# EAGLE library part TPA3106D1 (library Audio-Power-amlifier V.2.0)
40-W MONO CLASS-D AUDIO POWER AMPLIFIER
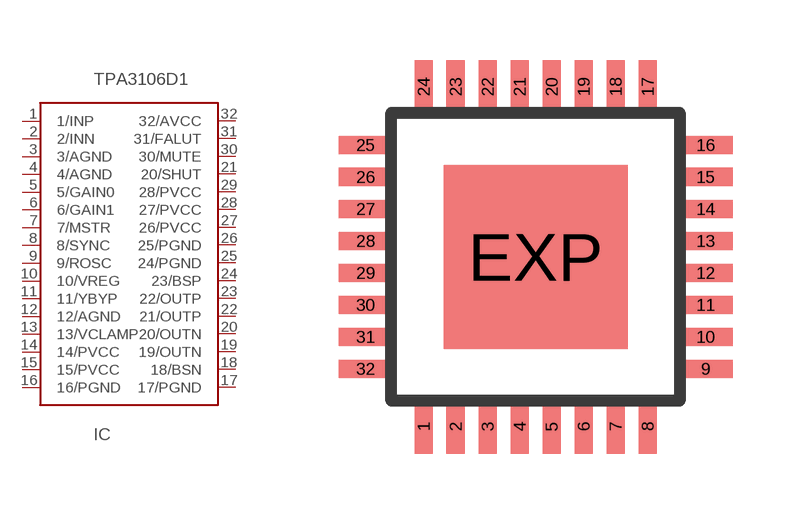
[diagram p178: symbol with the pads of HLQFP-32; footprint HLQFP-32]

Designator prefix IC

## TPA3106D1  [HLQFP-32]
1  1/INP  in
2  2/INN  in
3  3/AGND  pwr
4  4/AGND  pwr
5  5/GAIN0  in
6  6/GAIN1  in
7  7/MSTR  in
8  8/SYNC
9  9/ROSC
10  10/VREG  out
11  11/YBYP  out
12  12/AGND  pwr
13  13/VCLAMP  pwr
14  14/PVCC  pwr
15  15/PVCC  pwr
16  16/PGND  pwr
17  17/PGND  pwr
18  18/BSN
19  19/OUTN  out
20  20/OUTN  out
21  20/SHUT  in
22  21/OUTP  out
23  22/OUTP  out
24  23/BSP
25  24/PGND  pwr
26  25/PGND  pwr
27  26/PVCC  pwr
28  27/PVCC  pwr
29  28/PVCC  pwr
30  30/MUTE  in
31  31/FALUT  out
32  32/AVCC  pwr

## Footprint HLQFP-32 (pad centres in mm)
smd 0.45 x 1.35: 1 -2.8,-4.25; 2 -2,-4.25; 3 -1.2,-4.25; 4 -0.4,-4.25; 5 0.4,-4.25; 6 1.2,-4.25; 7 2,-4.25; 8 2.8,-4.25; 17 2.8,4.25; 18 2,4.25; 19 1.2,4.25; 20 0.4,4.25; 21 -0.4,4.25; 22 -1.2,4.25; 23 -2,4.25; 24 -2.8,4.25
smd 1.35 x 0.45: 9 4.25,-2.8; 10 4.25,-2; 11 4.25,-1.2; 12 4.25,-0.4; 13 4.25,0.4; 14 4.25,1.2; 15 4.25,2; 16 4.25,2.8; 25 -4.25,2.8; 26 -4.25,2; 27 -4.25,1.2; 28 -4.25,0.4; 29 -4.25,-0.4; 30 -4.25,-1.2; 31 -4.25,-2; 32 -4.25,-2.8
smd 4.6 x 4.6: EXP 0,0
